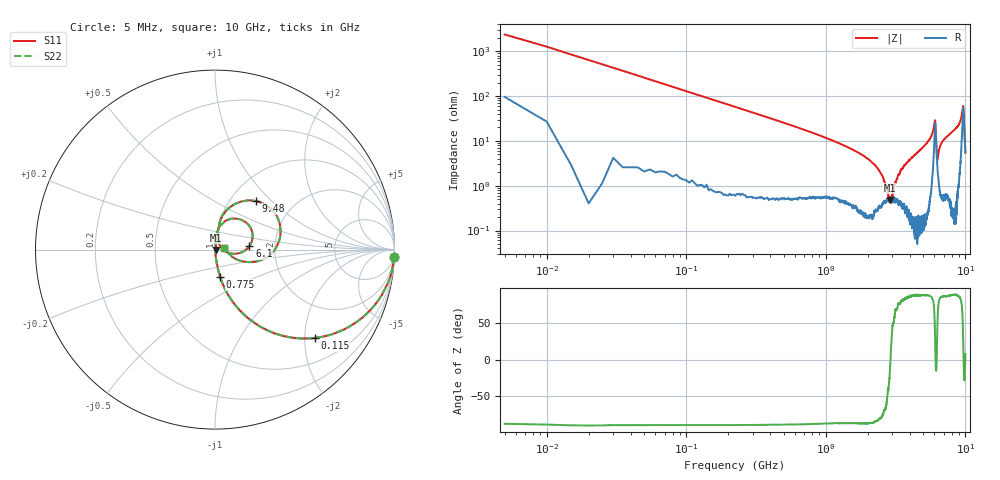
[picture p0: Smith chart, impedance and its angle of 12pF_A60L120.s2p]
! Amotech Co.,Ltd.
! http://www.amotech.co.kr/
! Part Number: A60L120
! These Parameters are Measured in Series Mode Connection
! Operation Temp=25[degC], DC Bias Voltage=0[V]
! Freq. Start=5[MHz] Stop=10[GHz], 2000[Steps]
! Date: Monday, July 14, 2020, 09:36:22
# GHZ S RI R 50.000000
!Freq.(Hz) S11(Real) S11(Imag) S21(Real) S21(Imag) S12(Real) S12(Imag) S22(Real) S22(Imag)
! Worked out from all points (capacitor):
!   2000 points, 5 MHz to 10 GHz, reference 50 ohm
!   read as one part in series: C = 12.4 pF near 55 MHz
!   lowest |Z| = 480 mohm at 2.86 GHz (marker M1)
!   series resonance near 2.906 GHz, so ESL is about 240 pH
!   S11 on the Smith chart (normalised r, x): 5 MHz: 3, -47; 115 MHz: 1.02, -2.24; 775 MHz: 1.01, -0.32; 6.1 GHz: 1.47, +0.06; 9.48 GHz: 1.31, +0.81; 10 GHz: 1.11, +0.02
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0.005  0.9965 -0.042  0.00347 0.042  0.00347 0.042  0.9965 -0.042
0.065  0.7953 -0.3983  0.2047 0.3983  0.2047 0.3983  0.7953 -0.3983
0.115  0.5551 -0.4919  0.4449 0.4919  0.4449 0.4919  0.5551 -0.4919
0.2  0.2956 -0.4517  0.7044 0.4517  0.7044 0.4517  0.2956 -0.4517
0.315  0.1457 -0.3465  0.8543 0.3465  0.8543 0.3465  0.1457 -0.3465
0.775  0.0294 -0.1524  0.9706 0.1524  0.9706 0.1524  0.0294 -0.1524
1.675  0.00637 -0.056  0.9936 0.056  0.9936 0.056  0.00637 -0.056
2.415  0.00401 -0.0212  0.996 0.0212  0.996 0.0212  0.00401 -0.0212
2.86  0.00431 -0.00206  0.9957 0.00206  0.9957 0.00206  0.00431 -0.00206
3.34  0.00443 0.0176  0.9956 -0.0176  0.9956 -0.0176  0.00443 0.0176
3.91  0.00361 0.0353  0.9964 -0.0353  0.9964 -0.0353  0.00361 0.0353
5.005  0.00654 0.0737  0.9935 -0.0737  0.9935 -0.0737  0.00654 0.0737
5.965  0.0997 0.1728  0.9003 -0.1728  0.9003 -0.1728  0.0997 0.1728
6.1  0.1918 0.0196  0.8082 -0.0196  0.8082 -0.0196  0.1918 0.0196
6.23  0.0472 -0.000449  0.9528 0.000449  0.9528 0.000449  0.0472 -0.000449
6.285  0.0292 0.0204  0.9708 -0.0204  0.9708 -0.0204  0.0292 0.0204
6.67  0.0127 0.0815  0.9873 -0.0815  0.9873 -0.0815  0.0127 0.0815
8.335  0.0314 0.1695  0.9686 -0.1695  0.9686 -0.1695  0.0314 0.1695
9.16  0.0847 0.2388  0.9153 -0.2388  0.9153 -0.2388  0.0847 0.2388
9.48  0.2276 0.2706  0.7724 -0.2706  0.7724 -0.2706  0.2276 0.2706
9.7  0.3265 -0.00829  0.6735 0.00829  0.6735 0.00829  0.3265 -0.00829
10  0.0517 0.00688  0.9483 -0.00688  0.9483 -0.00688  0.0517 0.00688
